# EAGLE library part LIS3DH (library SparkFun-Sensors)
ST Microelectronics LIS3DH 3-Axis &plusmn;2/4/8/16g SPI/I2C Accelerometer The LIS3DH is a three axis MEMS linear accelerometer in the "nano" family. It has a digital I2C/SPI serial interface which makes it ideal for using in embedded applications. The device also features ultra low-power operational modes that allow advanced power saving and smart sleep to wake-up functions, built in detections with interrupts, and auxiliary ADC inputs Datasheet-XXXX SparkFun Products SparkFun Triple Axis Accelerometer Breakout - LIS3DH (SEN-XXXXX) Triple Axis Accelerometer - LIS3DH (SEN-XXXXX)
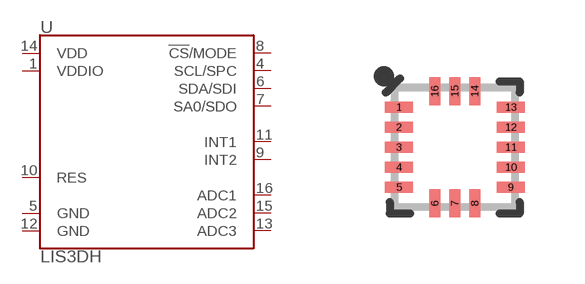
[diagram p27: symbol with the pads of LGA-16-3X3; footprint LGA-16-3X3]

Designator prefix U

## LIS3DH (PROD_ID: IC-13419; SF_ID: N/A)  [LGA-16-3X3]
1  VDDIO
4  SCL/SPC
5  GND
6  SDA/SDI
7  SA0/SDO
8  !CS!/MODE
9  INT2
10  RES
11  INT1
12  GND
13  ADC3
14  VDD
15  ADC2
16  ADC1

## Footprint LGA-16-3X3 (pad centres in mm)
16-Pin Land Grid Array (LGA) (3 x 3 mm) Datasheet Specifications: Pin Count: 16 Area: 3.0 x 3.0 x 1.0 mm Pitch: 0.5 mm Devices Using: LIS331 LIS3DH
smd 0.7 x 0.28: 1 -1.4,1; 2 -1.4,0.5; 3 -1.4,0; 4 -1.4,-0.5; 5 -1.4,-1; 9 1.4,-1; 10 1.4,-0.5; 11 1.4,0; 12 1.4,0.5; 13 1.4,1
smd 0.28 x 0.7: 6 -0.5,-1.4; 7 0,-1.4; 8 0.5,-1.4; 14 0.5,1.4; 15 0,1.4; 16 -0.5,1.4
